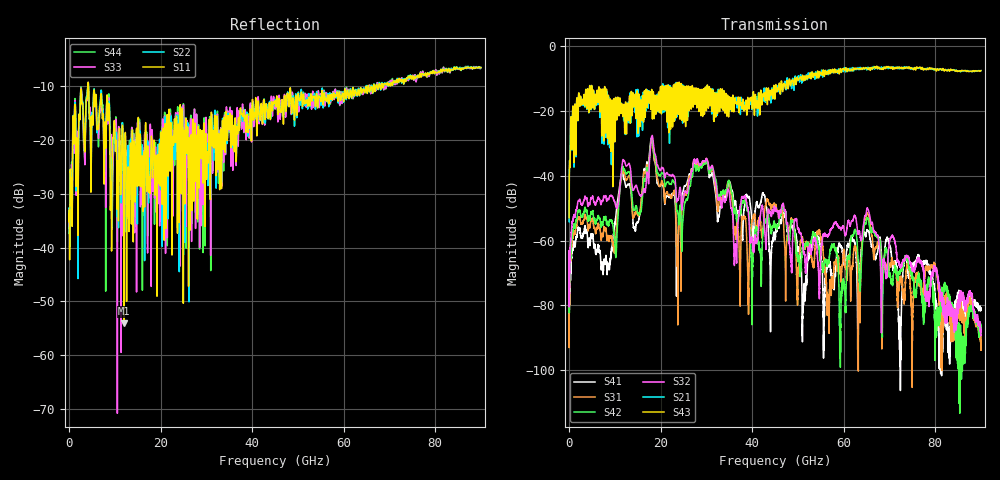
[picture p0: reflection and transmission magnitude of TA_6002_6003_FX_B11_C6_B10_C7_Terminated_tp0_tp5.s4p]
!Touchstone File created by Channel Assembly Engine (Version 2.0.0_Beta1)
!Current time:  2022 6/29 11:36:59
# Hz S RI R 50
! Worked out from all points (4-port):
!   9000 points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, 10 MHz to 90 GHz, reference 50 ohm
!   strongest paths, dB at 10 MHz, 22.51 GHz, 45.01 GHz, 67.51 GHz, 90 GHz:
!     S43: -52.9, -15.5, -15.9, -6.9, -7.5
!     S21: -54.2, -13.6, -13.7, -6.7, -7.5
!     S32: -67.9, -39.8, -50.5, -58.7, -89.1
!     S42: -67.3, -41.6, -55.9, -58.7, -88.7
!     S31: -67.6, -46.2, -49.3, -60.5, -93.8
!     S41: -76.0, -45.5, -59.8, -62.5, -81.5
!   lowest |S11| = -54.1 dB at 12.04 GHz (marker M1), VSWR 1.00, Z = 50.2 - j0.12 ohm
!   |S11| at or under -10 dB: start of sweep to 4.077 GHz; 4.259 GHz to 65.34 GHz (61.08 GHz wide, 176 % of centre); 65.47 GHz to 66.52 GHz (1.046 GHz wide, 1.59 % of centre)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
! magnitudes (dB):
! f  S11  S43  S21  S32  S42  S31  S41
! 10 MHz  -33.7  -52.9  -54.2  -67.9  -67.3  -67.6  -76.0
! 2.09 GHz  -17.9  -14.6  -15.1  -47.7  -50.9  -53.0  -56.5
! 8.63 GHz  -14.5  -15.7  -15.6  -47.4  -55.4  -59.6  -67.8
! 12.04 GHz  -54.1  -19.1  -19.4  -35.3  -37.9  -39.1  -41.0
! 42.47 GHz  -13.2  -15.5  -15.4  -51.9  -56.6  -55.1  -45.8
! 51.32 GHz  -12.1  -10.4  -10.5  -63.7  -62.2  -61.8  -74.4
! 90 GHz  -6.5  -7.5  -7.5  -89.1  -88.7  -93.8  -81.5
